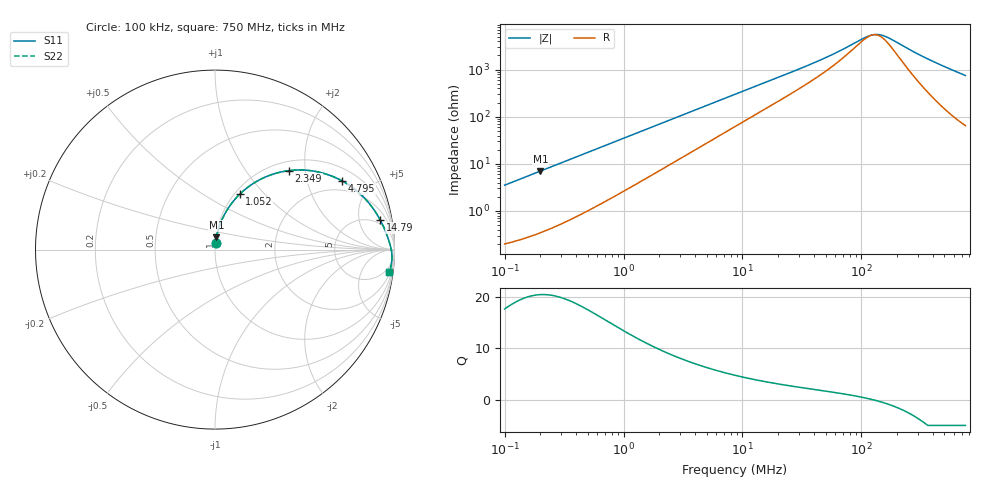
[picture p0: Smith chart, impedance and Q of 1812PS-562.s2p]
# MHz S MA R 50
!Freq  MagS11  AngS11  MagS21  AngS21  MagS12  AngS12  MagS22  AngS22
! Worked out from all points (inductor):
!   801 points, 100 kHz to 750 MHz, reference 50 ohm
!   read as one part in series: L = 5.59 uH near 104.6 kHz
!   highest Q = 20.4 at 199.7 kHz (marker M1), where L = 5.59 uH
!   self-resonance near 125 MHz
!   S11 on the Smith chart (normalised r, x): 100 kHz: 1.00, +0.07; 1.052 MHz: 1.06, +0.74; 2.349 MHz: 1.18, +1.63; 4.795 MHz: 1.52, +3.29; 14.79 MHz: 4, +10; 750 MHz: 2, -15
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0.1  0.03512 84.7  0.9974 -2.0  0.9974 -2.0  0.03512 84.7
0.199672  0.06982 83.2  0.9942 -4.0  0.9942 -4.0  0.06982 83.2
0.4457309  0.1534 78.0  0.9797 -8.8  0.9797 -8.8  0.1534 78.0
0.7120549  0.2389 72.5  0.9557 -13.8  0.9557 -13.8  0.2389 72.5
1.052077  0.3379 65.9  0.9158 -19.7  0.9158 -19.7  0.3379 65.9
1.437721  0.4348 59.3  0.8633 -25.7  0.8633 -25.7  0.4348 59.3
1.964725  0.5415 51.6  0.7878 -32.6  0.7878 -32.6  0.5415 51.6
2.348567  0.6028 46.9  0.7344 -36.8  0.7344 -36.8  0.6028 46.9
3.281842  0.7092 37.9  0.6195 -44.7  0.6195 -44.7  0.7092 37.9
4.795212  0.8044 28.5  0.4824 -52.6  0.4824 -52.6  0.8044 28.5
6.408366  0.8566 22.3  0.3855 -57.4  0.3855 -57.4  0.8566 22.3
8.660254  0.8946 17.0  0.299 -61.1  0.299 -61.1  0.8946 17.0
14.79225  0.9349 10.2  0.1841 -64.3  0.1841 -64.3  0.9349 10.2
38.60143  0.9664 3.7  0.07177 -60.3  0.07177 -60.3  0.9664 3.7
59.63657  0.9738 2.1  0.04408 -52.5  0.04408 -52.5  0.9738 2.1
101.863  0.9802 0.5  0.02178 -24.5  0.02178 -24.5  0.9802 0.5
117.7568  0.9816 0.2  0.0186 -8.1  0.0186 -8.1  0.9816 0.2
128.7469  0.9824 -0.1  0.01769 4.2  0.01769 4.2  0.9824 -0.1
140.7626  0.9831 -0.3  0.01773 17.2  0.01773 17.2  0.9831 -0.3
170.1501  0.9844 -0.8  0.0209 41.4  0.0209 41.4  0.9844 -0.8
347.4059  0.9869 -3.1  0.05559 74.8  0.05559 74.8  0.9869 -3.1
750  0.9802 -7.5  0.1306 77.6  0.1306 77.6  0.9802 -7.5
